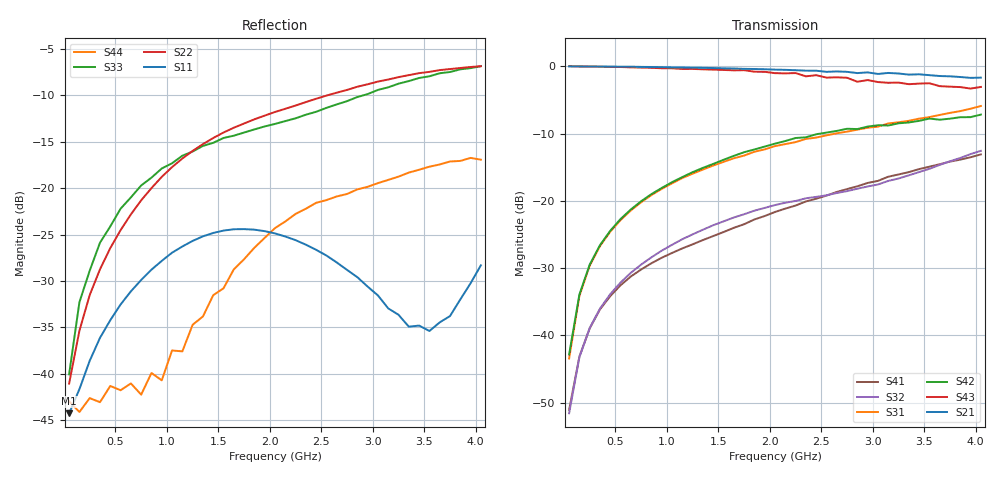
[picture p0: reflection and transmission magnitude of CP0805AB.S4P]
! Network Analyzer HP8720D.07.14 Serial No. US38111185
! 28 Apr 1999  02:06:29
! Frequency 	S11		S21		S31		S41		S12		S22		S23		S24		S13		S23		S33		S34		S14		S24		S34		S44
# HZ  S  DB R 50
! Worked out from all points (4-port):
!   41 points, 50 MHz to 4.05 GHz, reference 50 ohm
!   strongest paths, dB at 50 MHz, 1.05 GHz, 2.05 GHz, 3.05 GHz, 4.05 GHz:
!     S21: 0.0, -0.1, -0.5, -1.1, -1.7
!     S43: 0.0, -0.3, -1.0, -2.3, -3.1
!     S42: -42.8, -17.2, -11.5, -8.8, -7.2
!     S31: -43.5, -17.4, -11.9, -9.0, -5.9
!     S32: -51.6, -26.5, -20.6, -17.6, -12.6
!     S41: -51.1, -27.7, -21.7, -17.0, -13.1
!   lowest |S11| = -44.3 dB at 50 MHz (marker M1), VSWR 1.01, Z = 50.6 - j0.154 ohm
!   |S11| at or under -10 dB: start of sweep to end of sweep
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5e7  -44.27 -14.4  -0.01 -1.1  -44.29 85.0  -51.26 82.0
     0.00 -0.8  -41.07 46.1  -58.48 94.5  -45.64 87.7
     -43.45 90.1  -51.60 74.9  -40.06 40.6  -0.00 -1.6
     -51.09 73.9  -42.84 91.9  0.03 -1.2  -42.98 -9.8
1.5e8  -41.66 -58.6  0.00 -2.6  -34.08 86.9  -43.48 86.2
       0.00 -2.7  -35.37 63.5  -43.20 87.7  -33.92 86.6
       -34.12 86.1  -43.26 87.7  -32.29 65.8  -0.00 -4.0
       -43.15 86.0  -33.93 85.7  -0.02 -4.0  -44.12 -2.5
2.5e8  -38.60 -83.2  -0.01 -4.5  -29.65 84.8  -39.02 84.8
       -0.01 -4.5  -31.52 69.1  -38.88 86.1  -29.50 84.2
       -29.64 84.4  -38.91 85.8  -28.89 64.1  -0.03 -6.5
       -38.97 84.0  -29.48 84.3  -0.04 -6.7  -42.63 -31.8
7.5e8  -29.89 -152.0  -0.07 -13.1  -20.23 74.7  -30.17 75.9
       -0.08 -13.3  -21.31 65.7  -29.46 80.2  -20.09 73.3
       -20.21 74.6  -29.48 80.1  -19.70 48.0  -0.19 -19.4
       -30.20 75.6  -20.05 73.2  -0.18 -19.5  -42.25 -80.4
2.05e9  -24.88 134.1  -0.52 -36.1  -11.70 48.8  -21.45 68.6
        -0.48 -35.5  -11.79 -0.6  -20.41 61.3  -11.94 47.4
        -11.86 52.0  -20.63 64.3  -13.07 -6.9  -0.98 -52.5
        -21.65 71.4  -11.49 44.5  -1.01 -52.9  -24.30 159.6
3.55e9  -35.39 92.4  -1.28 -64.0  -7.00 20.8  -14.46 44.2
        -1.31 -62.9  -7.46 -75.0  -14.98 47.5  -7.88 19.8
        -7.54 27.9  -15.24 55.4  -7.94 -72.1  -1.94 -89.4
        -14.92 51.8  -7.76 10.7  -2.51 -90.1  -17.68 50.5
4.05e9  -28.31 70.0  -2.05 -72.6  -6.06 6.9  -13.36 27.4
        -1.67 -71.3  -6.85 -96.4  -13.17 33.4  -6.63 11.5
        -5.89 19.8  -12.56 46.5  -6.85 -99.3  -2.77 -107.5
        -13.09 42.1  -7.17 3.9  -3.06 -100.9  -16.93 18.7
